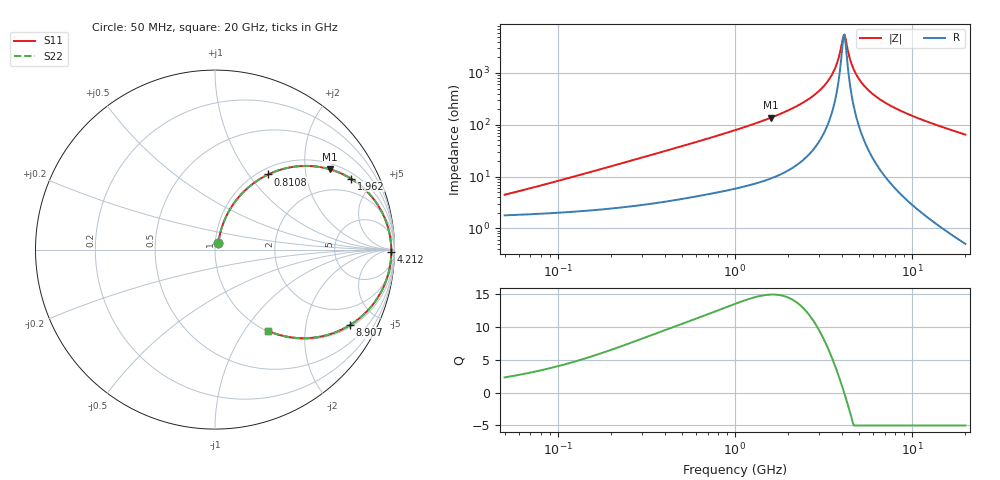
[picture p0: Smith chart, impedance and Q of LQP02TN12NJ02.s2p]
!Murata Part Number: LQP02TN12NJ02
!These Parameters are Measured in Series Mode Connection
!  o--[Z]--o
!Port1  Port2
!  o-------o
!Freq. Start=50[MHz] Stop=20[GHz], 401[Steps]
# Hz S RI R 50
!Freq.(Hz) S11(Real) S11(Imag) S21(Real) S21(Imag) S12(Real) S12(Imag) S22(Real) S22(Imag)
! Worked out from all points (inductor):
!   401 points, 50 MHz to 20 GHz, reference 50 ohm
!   read as one part in series: L = 12.8 nH near 69.52 MHz
!   highest Q = 14.9 at 1.591 GHz (marker M1), where L = 13.6 nH
!   self-resonance near 4.088 GHz
!   S11 on the Smith chart (normalised r, x): 50 MHz: 1.04, +0.08; 810.8 MHz: 1.10, +1.25; 1.962 GHz: 1.25, +3.67; 4.212 GHz: 75, -54; 8.907 GHz: 1.08, -3.53; 20 GHz: 1.01, -1.29
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5e7  0.0191 0.0393  0.9809 -0.0393  0.9809 -0.0393  0.0191 0.0393
1.364002e8  0.0318 0.1021  0.9682 -0.1021  0.9682 -0.1021  0.0318 0.1021
3.721004e8  0.0997 0.2498  0.9003 -0.2498  0.9003 -0.2498  0.0997 0.2498
5.575697e8  0.1767 0.3382  0.8233 -0.3382  0.8233 -0.3382  0.1767 0.3382
8.108264e8  0.2971 0.4188  0.7029 -0.4188  0.7029 -0.4188  0.2971 0.4188
1e9  0.3891 0.4518  0.6109 -0.4518  0.6109 -0.4518  0.3891 0.4518
1.590961e9  0.6411 0.4472  0.3589 -0.4472  0.3589 -0.4472  0.6411 0.4472
1.962148e9  0.7575 0.3955  0.2425 -0.3955  0.2425 -0.3955  0.7575 0.3955
2.728004e9  0.9052 0.2515  0.0948 -0.2515  0.0948 -0.2515  0.9052 0.2515
3.121702e9  0.9456 0.1754  0.0544 -0.1754  0.0544 -0.1754  0.9456 0.1754
3.466789e9  0.9671 0.1117  0.0329 -0.1117  0.0329 -0.1117  0.9671 0.1117
3.736399e9  0.9768 0.0646  0.0232 -0.0646  0.0232 -0.0646  0.9768 0.0646
4.087748e9  0.9822 0.00699  0.0178 -0.00699  0.0178 -0.00699  0.9822 0.00699
4.212059e9  0.9825 -0.0123  0.0175 0.0123  0.0175 0.0123  0.9825 -0.0123
4.472136e9  0.9806 -0.051  0.0194 0.051  0.0194 0.051  0.9806 -0.051
4.608136e9  0.9785 -0.0703  0.0215 0.0703  0.0215 0.0703  0.9785 -0.0703
5.041459e9  0.9675 -0.1275  0.0325 0.1275  0.0325 0.1275  0.9675 -0.1275
5.944466e9  0.9296 -0.2279  0.0704 0.2279  0.0704 0.2279  0.9296 -0.2279
7.442007e9  0.8438 -0.347  0.1562 0.347  0.1562 0.347  0.8438 -0.347
8.907419e9  0.7521 -0.4204  0.2479 0.4204  0.2479 0.4204  0.7521 -0.4204
1.295331e10  0.529 -0.4926  0.471 0.4926  0.471 0.4926  0.529 -0.4926
2e10  0.2949 -0.4521  0.7051 0.4521  0.7051 0.4521  0.2949 -0.4521
